PROGRAM MAIN
VAR
	fbKL6581			:	FB_KL6581;
	fbRec_RPS_Switch	:	FB_Rec_RPS_Switch;
	dwID				:	DWORD;
	stEnOceanSwitch		:	STR_EnOceanSwitch;
END_VAR

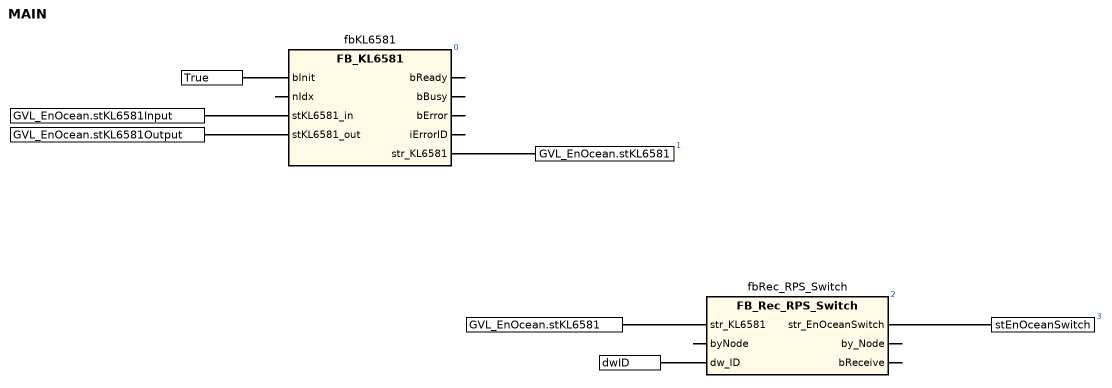
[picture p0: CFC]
fbKL6581(bInit := True, stKL6581_in := GVL_EnOcean.stKL6581Input, stKL6581_out := GVL_EnOcean.stKL6581Output); // FB_KL6581
GVL_EnOcean.stKL6581 := fbKL6581.str_KL6581;
fbRec_RPS_Switch(str_KL6581 := GVL_EnOcean.stKL6581, dw_ID := dwID); // FB_Rec_RPS_Switch
stEnOceanSwitch := fbRec_RPS_Switch.str_EnOceanSwitch;

END_PROGRAM
